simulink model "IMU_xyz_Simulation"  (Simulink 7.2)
settings: Solver=FixedStepDiscrete  StartTime=0.0  StopTime=110  FixedStep=.001  RelTol=1e-3
PreLoadFcn:
  | Script_Kalman
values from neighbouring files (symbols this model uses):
  Az = [1 -Ts ;0 1]    [Script_Kalman.m]
  Kz = 1e-3*[.4 ; -.04]    [Script_Kalman.m]
  Ts = .001    (= 0.001)    [Script_Kalman.m]
undefined symbols (not defined in the file or in its folder): DiscIntNeverNeededParam, float
libraries: simulink x40
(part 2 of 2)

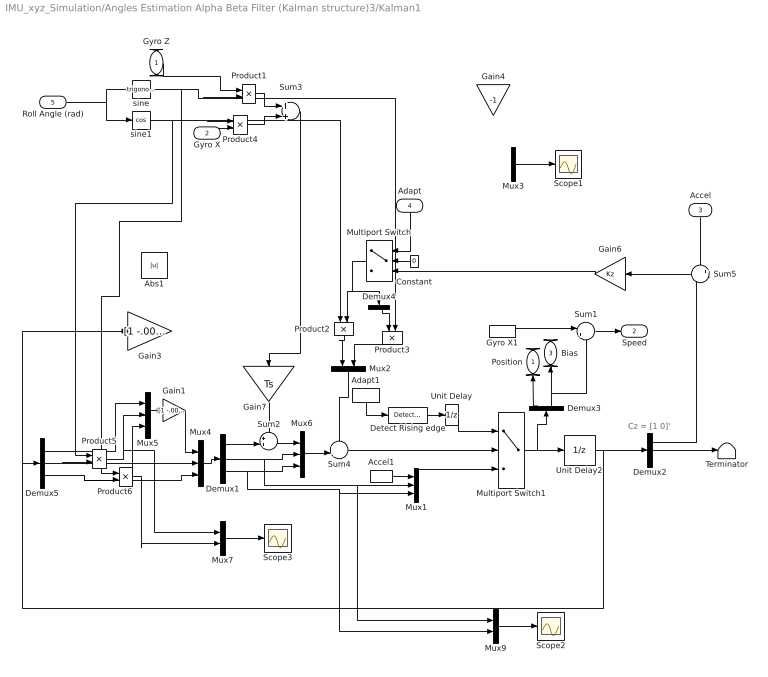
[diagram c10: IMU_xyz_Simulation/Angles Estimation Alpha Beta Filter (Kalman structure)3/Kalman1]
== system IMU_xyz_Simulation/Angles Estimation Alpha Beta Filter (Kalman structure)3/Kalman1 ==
  note: Cz = [1 0]'
  Gyro Z : Inport
  Gyro X : Inport  Port=2
  Accel : Inport  Orientation=down  Port=3
  Adapt : Inport  Orientation=down  Port=4
  Roll Angle (rad) : Inport  Port=5
  Abs1 : Abs  Orientation=down  OutDataType=sfix(16)  OutScaling=2^0
  Accel1 : InportShadow  Port=3  LatchByCopyingInsideSignal=off
  Adapt1 : InportShadow  Orientation=down  Port=4  LatchByCopyingInsideSignal=off
  Constant : Constant  Orientation=left  Value=0  OutDataType=sfix(16)  OutScaling=2^0
  Demux1 : Demux  Outputs=3
  Demux2 : Demux  Outputs=3
  Demux3 : Demux  Orientation=up  Outputs=3
  Demux4 : Demux  Orientation=down  Outputs=2
  Demux5 : Demux  Outputs=3
  Detect Rising edge : simulink/Logic and Bit Operations/Detect Increase  SystemSampleTime=-1  vinit=0
  Gain1 : Gain  Gain=[1 -.001 -.001]  Multiplication=Matrix(K*u)  ParameterDataType=sfix(16)  ParameterScaling=2^0  OutDataType=sfix(16)  OutScaling=2^0
  Gain3 : Gain  Gain=[1 -.001 -.001 ; 0 1 0 ; 0 0 1]  Multiplication=Matrix(K*u)  ParameterDataType=sfix(16)  ParameterScaling=2^0  OutDataType=sfix(16)  OutScaling=2^0
  Gain4 : Gain  Orientation=down  Gain=-1  Multiplication=Matrix(K*u)  ParameterDataType=sfix(16)  ParameterScaling=2^0  OutDataType=sfix(16)  OutScaling=2^0
  Gain6 : Gain  Orientation=left  Gain=Kz  Multiplication=Matrix(K*u)  ParameterDataType=sfix(16)  ParameterScaling=2^0  OutDataType=sfix(16)  OutScaling=2^0
  Gain7 : Gain  Orientation=down  Gain=Ts  Multiplication=Matrix(K*u)  ParameterDataType=sfix(16)  ParameterScaling=2^0  OutDataType=sfix(16)  OutScaling=2^0
  Gyro X1 : InportShadow  Port=2  LatchByCopyingInsideSignal=off
  Multiport Switch : MultiPortSwitch  Orientation=left  Inputs=2  zeroidx=on
  Multiport Switch1 : MultiPortSwitch  Inputs=2  zeroidx=on
  Mux{1,4..6} (4 alike) : Mux  Inputs=3
  Mux2 : Mux  Orientation=down  Inputs=2
  Mux3 : Mux  Inputs=2
  Mux7 : Mux  Inputs=2
  Mux9 : Mux  Inputs=2
  Product{1,4..6} (4 alike) : Product  OutDataType=sfix(16)  OutScaling=2^0
  Product2 : Product  Orientation=down  OutDataType=sfix(16)  OutScaling=2^0
  Product3 : Product  Orientation=down  OutDataType=sfix(16)  OutScaling=2^0
  Scope1 : Scope
  Scope2 : Scope
  Scope3 : Scope
  Sum1 : Sum  Inputs=|+-  OutDataType=sfix(16)  OutScaling=2^0
  Sum2 : Sum  Inputs=++|  OutDataType=sfix(16)  OutScaling=2^0
  Sum3 : Sum  OutDataType=sfix(16)  OutScaling=2^0
  Sum4 : Sum  Inputs=++|  OutDataType=sfix(16)  OutScaling=2^0
  Sum5 : Sum  Orientation=left  Inputs=+-  OutDataType=sfix(16)  OutScaling=2^0
  Terminator : Terminator
  Unit Delay : UnitDelay  SampleTime=-1
  Unit Delay2 : UnitDelay  X0=[0 0 0]  SampleTime=-1
  sine : Trigonometry
  sine1 : Trigonometry  Operator=cos
  Position : Outport  Orientation=up  OutDataType=sfix(16)  OutScaling=2^0
  Speed : Outport  Port=2  OutDataType=sfix(16)  OutScaling=2^0
  Bias : Outport  Orientation=up  Port=3  OutDataType=sfix(16)  OutScaling=2^0
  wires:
  Demux2/2 -> Terminator/1
  Mux1/1 -> Multiport Switch1/3
  Accel1/1 -> Mux1/1
  Adapt1/1 -> Detect Rising edge/1
  Sum4/1 -> Multiport Switch1/2
  Multiport Switch1/1 -> Unit Delay2/1, Demux3/1
  Detect Rising edge/1 -> Unit Delay/1
  Constant/1 -> Multiport Switch/2
  Gain6/1 -> Multiport Switch/3
  Adapt/1 -> Multiport Switch/1
  Demux2/1 -> Sum5/2
  Demux1/1 -> Sum2/2
  Sum2/1 -> Mux6/1
  Demux1/2 -> Mux6/2, Mux1/2, Mux9/1
  Mux6/1 -> Sum4/2
  Sum5/1 -> Gain6/1
  Gain7/1 -> Sum2/1
  Accel/1 -> Sum5/1
  Unit Delay/1 -> Multiport Switch1/1
  Unit Delay2/1 -> Demux2/1, Demux5/1, Gain3/1
  Demux3/1 -> Position/1
  Demux3/2 -> Bias/1, Sum1/2
  Sum1/1 -> Speed/1
  Roll Angle (rad)/1 -> sine/1, sine1/1
  sine1/1 -> Product4/1, Product2/1, Product5/1
  Gyro X/1 -> Product4/2
  Gyro Z/1 -> Product1/1
  sine/1 -> Product1/2, Product3/2, Product6/1
  Product1/1 -> Sum3/1
  Product4/1 -> Sum3/2
  Sum3/1 -> Gain7/1
  Multiport Switch/1 -> Product2/2, Demux4/1
  Gyro X1/1 -> Sum1/1
  Demux1/3 -> Mux6/3, Mux1/3, Mux9/2
  Product2/1 -> Mux2/1
  Mux2/1 -> Sum4/1
  Mux9/1 -> Scope2/1
  Demux4/2 -> Product3/1
  Mux3/1 -> Scope1/1
  Demux5/2 -> Product5/2, Mux4/2
  Demux5/3 -> Product6/2, Mux4/3
  Product6/1 -> Mux5/3, Mux7/2
  Product5/1 -> Mux5/2, Mux7/1
  Mux5/1 -> Gain1/1
  Demux5/1 -> Mux5/1
  Gain1/1 -> Mux4/1
  Mux4/1 -> Demux1/1
  Mux7/1 -> Scope3/1
  Product3/1 -> Mux2/2

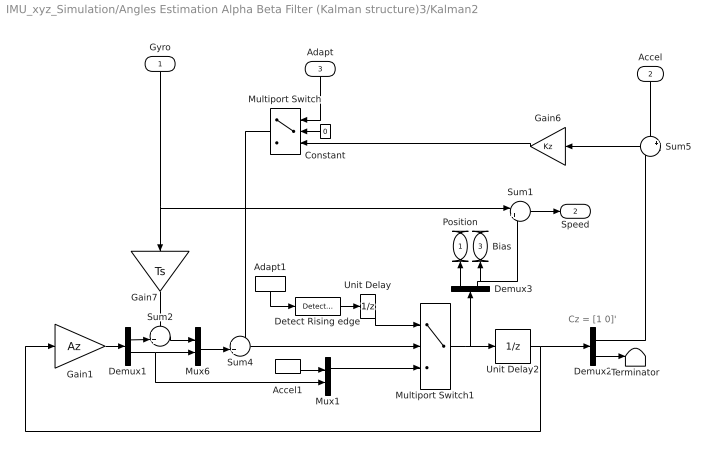
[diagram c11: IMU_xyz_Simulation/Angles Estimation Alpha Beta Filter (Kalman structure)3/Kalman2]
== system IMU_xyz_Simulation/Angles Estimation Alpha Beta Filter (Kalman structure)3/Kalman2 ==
  note: Cz = [1 0]'
  Gyro : Inport  Orientation=down
  Accel : Inport  Orientation=down  Port=2
  Adapt : Inport  Orientation=down  Port=3
  Accel1 : InportShadow  Port=2  LatchByCopyingInsideSignal=off
  Adapt1 : InportShadow  Orientation=down  Port=3  LatchByCopyingInsideSignal=off
  Constant : Constant  Orientation=left  Value=0  OutDataType=sfix(16)  OutScaling=2^0
  Demux1 : Demux  Outputs=2
  Demux2 : Demux  Outputs=2
  Demux3 : Demux  Orientation=up  Outputs=2
  Detect Rising edge : simulink/Logic and Bit Operations/Detect Increase  SystemSampleTime=-1  vinit=0
  Gain1 : Gain  Gain=Az  Multiplication=Matrix(K*u)  ParameterDataType=sfix(16)  ParameterScaling=2^0  OutDataType=sfix(16)  OutScaling=2^0
  Gain6 : Gain  Orientation=left  Gain=Kz  Multiplication=Matrix(K*u)  ParameterDataType=sfix(16)  ParameterScaling=2^0  OutDataType=sfix(16)  OutScaling=2^0
  Gain7 : Gain  Orientation=down  Gain=Ts  Multiplication=Matrix(K*u)  ParameterDataType=sfix(16)  ParameterScaling=2^0  OutDataType=sfix(16)  OutScaling=2^0
  Multiport Switch : MultiPortSwitch  Orientation=left  Inputs=2  zeroidx=on
  Multiport Switch1 : MultiPortSwitch  Inputs=2  zeroidx=on
  Mux1 : Mux  Inputs=2
  Mux6 : Mux  Inputs=2
  Sum1 : Sum  Inputs=|+-  OutDataType=sfix(16)  OutScaling=2^0
  Sum2 : Sum  Inputs=++|  OutDataType=sfix(16)  OutScaling=2^0
  Sum4 : Sum  Inputs=++|  OutDataType=sfix(16)  OutScaling=2^0
  Sum5 : Sum  Orientation=left  Inputs=+-  OutDataType=sfix(16)  OutScaling=2^0
  Terminator : Terminator
  Unit Delay : UnitDelay  SampleTime=-1
  Unit Delay2 : UnitDelay  SampleTime=-1
  Position : Outport  Orientation=up  OutDataType=sfix(16)  OutScaling=2^0
  Speed : Outport  Port=2  OutDataType=sfix(16)  OutScaling=2^0
  Bias : Outport  Orientation=up  Port=3  OutDataType=sfix(16)  OutScaling=2^0
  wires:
  Sum1/1 -> Speed/1
  Demux3/2 -> Sum1/2, Bias/1
  Demux3/1 -> Position/1
  Unit Delay2/1 -> Gain1/1, Demux2/1
  Unit Delay/1 -> Multiport Switch1/1
  Gyro/1 -> Sum1/1, Gain7/1
  Accel/1 -> Sum5/1
  Gain7/1 -> Sum2/1
  Sum5/1 -> Gain6/1
  Mux6/1 -> Sum4/2
  Demux1/2 -> Mux6/2, Mux1/2
  Sum2/1 -> Mux6/1
  Demux1/1 -> Sum2/2
  Gain1/1 -> Demux1/1
  Demux2/1 -> Sum5/2
  Multiport Switch/1 -> Sum4/1
  Adapt/1 -> Multiport Switch/1
  Gain6/1 -> Multiport Switch/3
  Constant/1 -> Multiport Switch/2
  Detect Rising edge/1 -> Unit Delay/1
  Multiport Switch1/1 -> Demux3/1, Unit Delay2/1
  Sum4/1 -> Multiport Switch1/2
  Adapt1/1 -> Detect Rising edge/1
  Accel1/1 -> Mux1/1
  Mux1/1 -> Multiport Switch1/3
  Demux2/2 -> Terminator/1

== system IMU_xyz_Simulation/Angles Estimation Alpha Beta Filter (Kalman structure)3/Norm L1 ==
  Accel Y : Inport
  Accel Z : Inport  Port=2
  Accel X : Inport  Port=3
  Abs : Abs
  Abs1 : Abs
  Abs2 : Abs
  Sum1 : Sum  OutDataType=sfix(16)  OutScaling=2^0
  Sum3 : Sum  OutDataType=sfix(16)  OutScaling=2^0
  abs(Y)+abs(Z) : Outport
  abs(X)+abs(Z) : Outport  Port=2
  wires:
  Sum1/1 -> abs(X)+abs(Z)/1
  Accel X/1 -> Abs2/1
  Abs2/1 -> Sum1/2
  Sum3/1 -> abs(Y)+abs(Z)/1
  Accel Z/1 -> Abs1/1
  Accel Y/1 -> Abs/1
  Abs1/1 -> Sum3/2, Sum1/1
  Abs/1 -> Sum3/1

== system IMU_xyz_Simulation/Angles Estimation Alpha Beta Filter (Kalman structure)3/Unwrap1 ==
  Estimated Angle : Inport
  Compare To Constant : simulink/Logic and Bit Operations/Compare To Constant  SystemSampleTime=-1  relop=>  const=180  LogicOutDataTypeMode=uint8  ZeroCross=off
  Compare To Constant1 : simulink/Logic and Bit Operations/Compare To Constant  SystemSampleTime=-1  relop=<  const=-180  LogicOutDataTypeMode=uint8  ZeroCross=off
  Compare To Zero : simulink/Logic and Bit Operations/Compare To Zero  SystemSampleTime=-1  relop=~=  LogicOutDataTypeMode=uint8  ZeroCross=off
  Difference : simulink/Discrete/Difference  SystemSampleTime=-1  ICPrevInput=0.0  OutMin=[]  OutMax=[]  OutDataType=sfix(16)  OutScaling=2^-10  DoSatur=off
  Discrete-Time Integrator : DiscreteIntegrator  gainval=1000  SampleTime=-1  OutDataType=sfix(16)  OutScaling=2^0  ICPrevOutput=DiscIntNeverNeededParam  ICPrevScaledInput=DiscIntNeverNeededParam
  Logical Operator : Logic  Orientation=up  Operator=NOR  AllPortsSameDT=off  OutDataTypeMode=boolean  OutDataTypeStr=boolean
  Lookup Table : Lookup  Orientation=left  InputValues=[-500 -195 195]  Table=[+360 0 -360]  LookUpMeth=Use Input Below  OutDataType=sfix(16)  OutScaling=2^0
  Merge : Merge  Inputs=3
  Sum2 : Sum  OutDataType=sfix(16)  OutScaling=2^0
  unwrap : Subsystem  TreatAsAtomicUnit=on
  unwrap1 : Subsystem  TreatAsAtomicUnit=on
  unwrap2 : Subsystem  TreatAsAtomicUnit=on
  unwrap angle : Outport
  Wrap : Outport  Port=2
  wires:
  Discrete-Time Integrator/1 -> unwrap angle/1, Lookup Table/1
  Estimated Angle/1 -> Difference/1
  unwrap1/1(Out1) -> Merge/3
  unwrap/1(Out1) -> Merge/2
  unwrap2/1(Out1) -> Merge/1
  Logical Operator/1 -> unwrap2/Enable
  Compare To Constant1/1 -> Logical Operator/2, unwrap1/Enable
  Compare To Constant/1 -> unwrap/Enable, Logical Operator/1
  Difference/1 -> unwrap2/1(In1), unwrap1/1(In1), Compare To Constant1/1, unwrap/1(In1), Compare To Constant/1
  Sum2/1 -> Discrete-Time Integrator/1
  Merge/1 -> Sum2/2
  Lookup Table/1 -> Sum2/1, Compare To Zero/1
  Compare To Zero/1 -> Wrap/1

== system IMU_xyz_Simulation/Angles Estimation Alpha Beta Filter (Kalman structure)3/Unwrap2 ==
  Estimated Angle : Inport
  Compare To Constant : simulink/Logic and Bit Operations/Compare To Constant  SystemSampleTime=-1  relop=>  const=180  LogicOutDataTypeMode=uint8  ZeroCross=off
  Compare To Constant1 : simulink/Logic and Bit Operations/Compare To Constant  SystemSampleTime=-1  relop=<  const=-180  LogicOutDataTypeMode=uint8  ZeroCross=off
  Compare To Zero : simulink/Logic and Bit Operations/Compare To Zero  SystemSampleTime=-1  relop=~=  LogicOutDataTypeMode=uint8  ZeroCross=off
  Difference : simulink/Discrete/Difference  SystemSampleTime=-1  ICPrevInput=0.0  OutMin=[]  OutMax=[]  OutDataType=sfix(16)  OutScaling=2^-10  DoSatur=off
  Discrete-Time Integrator : DiscreteIntegrator  gainval=1000  SampleTime=-1  OutDataType=sfix(16)  OutScaling=2^0  ICPrevOutput=DiscIntNeverNeededParam  ICPrevScaledInput=DiscIntNeverNeededParam
  Logical Operator : Logic  Orientation=up  Operator=NOR  AllPortsSameDT=off  OutDataTypeMode=boolean  OutDataTypeStr=boolean
  Lookup Table : Lookup  Orientation=left  InputValues=[-500 -195 195]  Table=[+360 0 -360]  LookUpMeth=Use Input Below  OutDataType=sfix(16)  OutScaling=2^0
  Merge : Merge  Inputs=3
  Sum2 : Sum  OutDataType=sfix(16)  OutScaling=2^0
  unwrap : Subsystem  TreatAsAtomicUnit=on
  unwrap1 : Subsystem  TreatAsAtomicUnit=on
  unwrap2 : Subsystem  TreatAsAtomicUnit=on
  unwrap angle : Outport
  Wrap : Outport  Port=2
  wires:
  Compare To Zero/1 -> Wrap/1
  Lookup Table/1 -> Compare To Zero/1, Sum2/1
  Merge/1 -> Sum2/2
  Sum2/1 -> Discrete-Time Integrator/1
  Difference/1 -> Compare To Constant/1, unwrap/1(In1), Compare To Constant1/1, unwrap1/1(In1), unwrap2/1(In1)
  Compare To Constant/1 -> Logical Operator/1, unwrap/Enable
  Compare To Constant1/1 -> unwrap1/Enable, Logical Operator/2
  Logical Operator/1 -> unwrap2/Enable
  unwrap2/1(Out1) -> Merge/1
  unwrap/1(Out1) -> Merge/2
  unwrap1/1(Out1) -> Merge/3
  Estimated Angle/1 -> Difference/1
  Discrete-Time Integrator/1 -> Lookup Table/1, unwrap angle/1

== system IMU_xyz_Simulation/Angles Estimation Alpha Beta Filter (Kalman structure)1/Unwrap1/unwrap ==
  In1 : Inport  OutDataType=sfix(16)  OutScaling=2^0
  Enable : EnablePort
  Bias2 : Constant  Value=-360  OutDataType=sfix(16)  OutScaling=2^0
  Sum2 : Sum  OutDataType=sfix(16)  OutScaling=2^0
  Out1 : Outport  OutDataType=sfix(16)  OutScaling=2^0
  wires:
  Bias2/1 -> Sum2/2
  Sum2/1 -> Out1/1
  In1/1 -> Sum2/1

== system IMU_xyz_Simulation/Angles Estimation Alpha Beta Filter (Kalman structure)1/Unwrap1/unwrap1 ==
  In1 : Inport  OutDataType=sfix(16)  OutScaling=2^0
  Enable : EnablePort
  Bias2 : Constant  Value=360  OutDataType=sfix(16)  OutScaling=2^0
  Sum2 : Sum  OutDataType=sfix(16)  OutScaling=2^0
  Out1 : Outport  OutDataType=sfix(16)  OutScaling=2^0
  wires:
  Sum2/1 -> Out1/1
  Bias2/1 -> Sum2/2
  In1/1 -> Sum2/1

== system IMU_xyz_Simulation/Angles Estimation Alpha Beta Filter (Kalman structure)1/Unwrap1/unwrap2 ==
  In1 : Inport  OutDataType=sfix(16)  OutScaling=2^0
  Enable : EnablePort
  Out1 : Outport  OutDataType=sfix(16)  OutScaling=2^0
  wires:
  In1/1 -> Out1/1

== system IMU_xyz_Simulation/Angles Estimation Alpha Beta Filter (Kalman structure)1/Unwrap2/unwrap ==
  In1 : Inport  OutDataType=sfix(16)  OutScaling=2^0
  Enable : EnablePort
  Bias2 : Constant  Value=-360  OutDataType=sfix(16)  OutScaling=2^0
  Sum2 : Sum  OutDataType=sfix(16)  OutScaling=2^0
  Out1 : Outport  OutDataType=sfix(16)  OutScaling=2^0
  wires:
  In1/1 -> Sum2/1
  Sum2/1 -> Out1/1
  Bias2/1 -> Sum2/2

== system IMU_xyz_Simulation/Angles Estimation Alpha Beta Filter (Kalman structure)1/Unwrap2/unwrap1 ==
  In1 : Inport  OutDataType=sfix(16)  OutScaling=2^0
  Enable : EnablePort
  Bias2 : Constant  Value=360  OutDataType=sfix(16)  OutScaling=2^0
  Sum2 : Sum  OutDataType=sfix(16)  OutScaling=2^0
  Out1 : Outport  OutDataType=sfix(16)  OutScaling=2^0
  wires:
  In1/1 -> Sum2/1
  Bias2/1 -> Sum2/2
  Sum2/1 -> Out1/1

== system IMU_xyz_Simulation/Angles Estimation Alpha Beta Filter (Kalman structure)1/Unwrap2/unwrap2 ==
  In1 : Inport  OutDataType=sfix(16)  OutScaling=2^0
  Enable : EnablePort
  Out1 : Outport  OutDataType=sfix(16)  OutScaling=2^0
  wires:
  In1/1 -> Out1/1

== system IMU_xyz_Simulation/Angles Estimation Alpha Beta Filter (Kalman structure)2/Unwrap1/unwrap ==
  In1 : Inport  OutDataType=sfix(16)  OutScaling=2^0
  Enable : EnablePort
  Bias2 : Constant  Value=-360  OutDataType=sfix(16)  OutScaling=2^0
  Sum2 : Sum  OutDataType=sfix(16)  OutScaling=2^0
  Out1 : Outport  OutDataType=sfix(16)  OutScaling=2^0
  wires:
  In1/1 -> Sum2/1
  Sum2/1 -> Out1/1
  Bias2/1 -> Sum2/2

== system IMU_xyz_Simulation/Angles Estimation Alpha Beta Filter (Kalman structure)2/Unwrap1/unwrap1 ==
  In1 : Inport  OutDataType=sfix(16)  OutScaling=2^0
  Enable : EnablePort
  Bias2 : Constant  Value=360  OutDataType=sfix(16)  OutScaling=2^0
  Sum2 : Sum  OutDataType=sfix(16)  OutScaling=2^0
  Out1 : Outport  OutDataType=sfix(16)  OutScaling=2^0
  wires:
  In1/1 -> Sum2/1
  Bias2/1 -> Sum2/2
  Sum2/1 -> Out1/1

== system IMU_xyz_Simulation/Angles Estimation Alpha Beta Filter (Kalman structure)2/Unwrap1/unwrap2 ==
  In1 : Inport  OutDataType=sfix(16)  OutScaling=2^0
  Enable : EnablePort
  Out1 : Outport  OutDataType=sfix(16)  OutScaling=2^0
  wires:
  In1/1 -> Out1/1

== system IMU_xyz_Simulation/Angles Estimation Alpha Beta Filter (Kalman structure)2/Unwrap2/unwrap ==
  In1 : Inport  OutDataType=sfix(16)  OutScaling=2^0
  Enable : EnablePort
  Bias2 : Constant  Value=-360  OutDataType=sfix(16)  OutScaling=2^0
  Sum2 : Sum  OutDataType=sfix(16)  OutScaling=2^0
  Out1 : Outport  OutDataType=sfix(16)  OutScaling=2^0
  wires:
  Bias2/1 -> Sum2/2
  Sum2/1 -> Out1/1
  In1/1 -> Sum2/1

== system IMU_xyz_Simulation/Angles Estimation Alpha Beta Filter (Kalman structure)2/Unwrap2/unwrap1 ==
  In1 : Inport  OutDataType=sfix(16)  OutScaling=2^0
  Enable : EnablePort
  Bias2 : Constant  Value=360  OutDataType=sfix(16)  OutScaling=2^0
  Sum2 : Sum  OutDataType=sfix(16)  OutScaling=2^0
  Out1 : Outport  OutDataType=sfix(16)  OutScaling=2^0
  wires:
  Sum2/1 -> Out1/1
  Bias2/1 -> Sum2/2
  In1/1 -> Sum2/1

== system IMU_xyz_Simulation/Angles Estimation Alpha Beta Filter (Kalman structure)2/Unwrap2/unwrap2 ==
  In1 : Inport  OutDataType=sfix(16)  OutScaling=2^0
  Enable : EnablePort
  Out1 : Outport  OutDataType=sfix(16)  OutScaling=2^0
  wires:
  In1/1 -> Out1/1

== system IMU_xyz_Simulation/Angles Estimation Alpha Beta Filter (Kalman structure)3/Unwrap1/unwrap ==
  In1 : Inport  OutDataType=sfix(16)  OutScaling=2^0
  Enable : EnablePort
  Bias2 : Constant  Value=-360  OutDataType=sfix(16)  OutScaling=2^0
  Sum2 : Sum  OutDataType=sfix(16)  OutScaling=2^0
  Out1 : Outport  OutDataType=sfix(16)  OutScaling=2^0
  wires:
  Bias2/1 -> Sum2/2
  Sum2/1 -> Out1/1
  In1/1 -> Sum2/1

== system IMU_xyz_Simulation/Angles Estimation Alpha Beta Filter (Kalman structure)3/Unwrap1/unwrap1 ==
  In1 : Inport  OutDataType=sfix(16)  OutScaling=2^0
  Enable : EnablePort
  Bias2 : Constant  Value=360  OutDataType=sfix(16)  OutScaling=2^0
  Sum2 : Sum  OutDataType=sfix(16)  OutScaling=2^0
  Out1 : Outport  OutDataType=sfix(16)  OutScaling=2^0
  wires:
  Sum2/1 -> Out1/1
  Bias2/1 -> Sum2/2
  In1/1 -> Sum2/1

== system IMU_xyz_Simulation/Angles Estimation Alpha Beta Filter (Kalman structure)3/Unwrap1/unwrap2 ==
  In1 : Inport  OutDataType=sfix(16)  OutScaling=2^0
  Enable : EnablePort
  Out1 : Outport  OutDataType=sfix(16)  OutScaling=2^0
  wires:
  In1/1 -> Out1/1

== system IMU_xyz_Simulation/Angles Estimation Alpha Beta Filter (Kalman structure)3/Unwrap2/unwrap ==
  In1 : Inport  OutDataType=sfix(16)  OutScaling=2^0
  Enable : EnablePort
  Bias2 : Constant  Value=-360  OutDataType=sfix(16)  OutScaling=2^0
  Sum2 : Sum  OutDataType=sfix(16)  OutScaling=2^0
  Out1 : Outport  OutDataType=sfix(16)  OutScaling=2^0
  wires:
  In1/1 -> Sum2/1
  Sum2/1 -> Out1/1
  Bias2/1 -> Sum2/2

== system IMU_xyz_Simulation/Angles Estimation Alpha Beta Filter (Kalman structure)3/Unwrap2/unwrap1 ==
  In1 : Inport  OutDataType=sfix(16)  OutScaling=2^0
  Enable : EnablePort
  Bias2 : Constant  Value=360  OutDataType=sfix(16)  OutScaling=2^0
  Sum2 : Sum  OutDataType=sfix(16)  OutScaling=2^0
  Out1 : Outport  OutDataType=sfix(16)  OutScaling=2^0
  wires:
  In1/1 -> Sum2/1
  Bias2/1 -> Sum2/2
  Sum2/1 -> Out1/1

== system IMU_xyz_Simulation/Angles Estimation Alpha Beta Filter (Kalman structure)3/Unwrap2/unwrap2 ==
  In1 : Inport  OutDataType=sfix(16)  OutScaling=2^0
  Enable : EnablePort
  Out1 : Outport  OutDataType=sfix(16)  OutScaling=2^0
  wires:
  In1/1 -> Out1/1
